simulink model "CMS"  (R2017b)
settings: Solver=FixedStepDiscrete  StartTime=0.0  StopTime=10.0  FixedStep=0.01  RelTol=1e-3  EnableMultiTasking=on
undefined symbols (not defined in the file): ASWTYPE_FALSE, ASWTYPE_TRUE, CcCMS_CANSendDelay_ms, CcCMS_ChrgMaxPackVoltLimt_V, CcCMS_PeakVoltCh_V, CcCMS_PeakVoltDisCh_V, CcSOC_DispSOCHighThrhd_pct, CMS09D_RUNTIME_MS, CMS_CONST0_NUMB, CMS_CONST1000_NUMB, CMS_CONST100_NUMB, CMS_CONST1_NUMB, CMS_CONST2047_NUMB, CMS_CONST2_NUMB, CMS_CONST3_NUMB, CMS_CONST4_NUMB, CMS_CONST5_NUMB, CMS_CONST6_NUMB, CMS_CONST7_NUMB, CMS_CONSTF1_NUMB, Enum_ACCACChrgState, Enum_CMSACChgMode, Enum_CMSBmsSelfChk, Enum_CMSBmsSt, Enum_CMSChgMode, Enum_CMSDCChgMode, Enum_CMSHVBatFltSevrtyStat, Enum_CMSHVConnSt, Enum_CMSPreThmMode, Enum_CMSPreThmReq, Enum_CMSThmPropagation, Enum_CTCCtrCtlConnMode, Enum_CTCCtrCtlState, Enum_DCCDCChrgState, Enum_DCCDCConnSt, Enum_ISOHVIsoFltLevel, Enum_MSMBMUState, Enum_ODPCCState, Enum_VDPPreThmEna
libraries: AIWAYS_Powertrain_BMS_lib x148
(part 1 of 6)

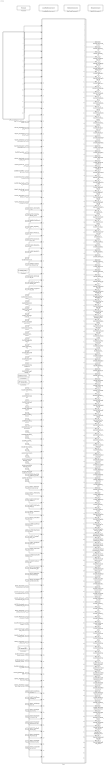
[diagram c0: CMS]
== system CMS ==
  GeCTC_CtrCtlState_enum : Inport
  GbCTC_NegCtlState_flg : Inport  Port=2
  GbCTC_PosCtlState_flg : Inport  Port=3
  GbCTC_DCPosChrgCtlState_flg : Inport  Port=4
  GbCTC_DCNegChrgCtlState_flg : Inport  Port=5
  GcHDP_PackVolt_V : Inport  Port=6
  GbCTC_PreChrgCtlState_flg : Inport  Port=7
  GcHDP_PackCrnt_A : Inport  Port=8
  GbWSM_Kl15WkUpPrs_flg : Inport  Port=9
  GcCDP_MinCellVolt_mV : Inport  Port=10
  GcCDP_MaxCellVolt_mV : Inport  Port=11
  GbACC_ObcChrgCmd_flg : Inport  Port=12
  GcACC_ACChrgVoltRqst_V : Inport  Port=13
  GcACC_ACChrgCrntRqst_A : Inport  Port=14
  GbACC_ACChrgRqst_flg : Inport  Port=15
  GeCTC_CtrCtlConnMode_enum : Inport  Port=16
  GbMSM_SelfCheck_flg : Inport  Port=17
  GcSOC_DispSOC_pct : Inport  Port=18
  GbISP_TFHvilLFlt_flg : Inport  Port=19
  GbFTC_OpenContactor_flg : Inport  Port=20
  GcSOH_PackSOH_pct : Inport  Port=21
  GcSOC_PackSOC_pct : Inport  Port=22
  GcHDP_HallCrnt_A : Inport  Port=23
  GbMSM_SelfChckMaxTiReach_flg : Inport  Port=24
  GbDCC_DCChrgRqst_flg : Inport  Port=25
  GcSOP_DischrgConstPwr_kW : Inport  Port=26
  GcSOP_ChrgConstPwr_kW : Inport  Port=27
  GcISO_HVIsoValue_kohm : Inport  Port=28
  GeODP_ObcCcSt_enum : Inport  Port=29
  GbDCC_DCChrgFinish_flg : Inport  Port=30
  GbACC_ACChrgFinish_flg : Inport  Port=31
  GeACC_ACChrgState_enum : Inport  Port=32
  GeDCC_DCConnSt_enum : Inport  Port=33
  GeLDP_CC2St_enum : Inport  Port=34
  GcCDP_AvgCellTemp_C : Inport  Port=35
  GbISO_IsoForbid_flg : Inport  Port=36
  GcCDP_MaxCellTemp_C : Inport  Port=37
  GcCDP_MinCellTemp_C : Inport  Port=38
  GcDCS_3072ChrgVoltReq_V : Inport  Port=39
  GcDCC_DCChrgCrntRqst_A : Inport  Port=40
  GcLDP_lntWtTemp_C : Inport  Port=41
  GcLDP_OutWtTemp_C : Inport  Port=42
  GcBTM_CoolPwrReq_W : Inport  Port=43
  GcBTM_HeatPwrReq_W : Inport  Port=44
  GeBTM_CoolReq_enum : Inport  Port=45
  GeBTM_HeatReq_enum : Inport  Port=46
  GbODP_V2XDischrgCmd_flg : Inport  Port=47
  GeMSM_BMUState_enum : Inport  Port=48
  GcHDP_FuseVolt_V : Inport  Port=49
  GbADP_DischgReq_flg : Inport  Port=50
  GcHDP_PosCtlVolt_V : Inport  Port=51
  GcCDP_MaxCellVoltNumb_numb : Inport  Port=52
  GcCDP_MinCellVoltNumb_numb : Inport  Port=53
  GcCDP_MaxCellTempNumb_numb : Inport  Port=54
  GcCDP_MinCellTempNumb_numb : Inport  Port=55
  GbWSM_DCWkUpPrs_flg : Inport  Port=56
  GbACC_PreThmObcChrgCmd_flg : Inport  Port=57
  GbACC_PreThmRqst_flg : Inport  Port=58
  GcACC_PreThmCrntRqst_A : Inport  Port=59
  GcACC_PreThmVoltRqst_V : Inport  Port=60
  GbACC_PreHeatPrmt_flg : Inport  Port=61
  GbFTC_PowerDown_flg : Inport  Port=62
  GcBTM_CoolTempReq_C : Inport  Port=63
  GcBTM_HeatTempReq_C : Inport  Port=64
  GcACC_ChrgingTiRem_min : Inport  Port=65
  GcDCC_ChrgingTiRem_min : Inport  Port=66
  GeVDP_PreThmEna_enum : Inport  Port=67
  GcSOP_DischrgPwr_kW : Inport  Port=68
  GcSOP_ChrgPwr_kW : Inport  Port=69
  GbFTC_DischrgPwrLimitLevel3_flg : Inport  Port=70
  GbFTC_RegenPwrLimitLevel3_flg : Inport  Port=71
  GbFTC_DischrgPwrLimitLevel2_flg : Inport  Port=72
  GbFTC_RegenPwrLimitLevel2_flg : Inport  Port=73
  GbFTC_DCChrgCurrLimitLevel2_flg : Inport  Port=74
  GbFTC_ACChrgCurrLimitLevel2_flg : Inport  Port=75
  GbFTC_DischrgPwrLimitLevel1_flg : Inport  Port=76
  GbFTC_RegenPwrLimitLevel1_flg : Inport  Port=77
  GcCDP_MaxBusbarTemp_C : Inport  Port=78
  GcCDP_MinBusbarTemp_C : Inport  Port=79
  GeDCC_DCChrgState_enum : Inport  Port=80
  GeLDP_ChrgGunConnSt_enum : Inport  Port=81
  GbISP_TFThmRnwyfDet_flg : Inport  Port=82
  GcUDS_CellTempNumb_numb : Inport  Port=83
  GcUDS_BusbarTempNumb_numb : Inport  Port=84
  GcUDS_CellVoltNum_numb : Inport  Port=85
  GcUDS_BatEnergy_kWh : Inport  Port=86
  GbACC_HoldTempPrmt_flg : Inport  Port=87
  GbACC_HoldTempObcChrgCmd_flg : Inport  Port=88
  GcACC_HoldTempVoltRqst_V : Inport  Port=89
  GcACC_HoldTempCrntRqst_A : Inport  Port=90
  GbACC_HoldTempRqst_flg : Inport  Port=91
  GbISP_TFIsoResFltLevel2_flg : Inport  Port=92
  GbISP_TFIsoDCResFltLevel2_flg : Inport  Port=93
  GbISP_TFIsoHVoffResFltLevel2_flg : Inport  Port=94
  GbISP_TFIsoResFltLevel1_flg : Inport  Port=95
  GbISP_TFIsoDCResFltLevel1_flg : Inport  Port=96
  GbISP_TFIsoHVoffResFltLevel1_flg : Inport  Port=97
  GbFTC_Level1FltReaction_flg : Inport  Port=98
  CMS : Subsystem
  CMS_Schedule : Stateflow chart  TreatAsAtomicUnit=on
  Constant : Constant  Value=1*ones(112,1)  OutDataTypeStr=boolean
  Constant1 : Constant  Value=25*ones(48,1)  OutDataTypeStr=single
  Constant2 : Constant  Value=25*ones(48,1)  OutDataTypeStr=single
  Constant3 : Constant  Value=4000*ones(112,1)  OutDataTypeStr=uint16
  LoadMptEnvironment : AIWAYS_Powertrain_BMS_lib/Config/LoadMptEnvironment  ProjectName=Comm  SuppierID=NewPlatformUAES
  MptA2LGenerate1 : AIWAYS_Powertrain_BMS_lib/Config/MptA2LGenerate  SystemSampleTime=-1
  MptCodeGenerate1 : AIWAYS_Powertrain_BMS_lib/Config/MptCodeGenerate  SystemSampleTime=-1
  Revision : AIWAYS_Powertrain_BMS_lib/Config/Revision  curVersion='M100C100'  newVersion='M100C100'
  GeCMS_HVConnSt_enum : Outport
  GbCMS_NegCtlSt_flg : Outport  Port=2
  GbCMS_PosCtlSt_flg : Outport  Port=3
  GbCMS_ChrgPosCtlSt_flg : Outport  Port=4
  GbCMS_ChrgNegCtlSt_flg : Outport  Port=5
  GeCMS_RelStuckClosed_enum : Outport  Port=6
  GcCMS_PackVolt_V : Outport  Port=7
  GbCMS_PreChrgCtlSt_flg : Outport  Port=8
  GcCMS_BattCurr_A : Outport  Port=9
  GbCMS_Kl15WkUp_flg : Outport  Port=10
  GbCMS_ThmRunAway_flg : Outport  Port=11
  GcCMS_CoolTempIn_C : Outport  Port=12
  GcCMS_CoolTempOut_C : Outport  Port=13
  GcCMS_CoolPwrReq_W : Outport  Port=14
  GcCMS_HeatPwrReq_W : Outport  Port=15
  GeCMS_CoolReq_enum : Outport  Port=16
  GeCMS_HeatReq_enum : Outport  Port=17
  GcCMS_PeakCurrDisCh_A : Outport  Port=18
  GcCMS_PeakCurrCh_A : Outport  Port=19
  GcCMS_PeakVoltDisCh_V : Outport  Port=20
  GcCMS_PeakVoltCh_V : Outport  Port=21
  GeCMS_Thm_propagat_enum : Outport  Port=22
  GcCMS_ClntTgtTemp_C : Outport  Port=23
  GcCMS_HtTgtTemp_C : Outport  Port=24
  GcCMS_MaxCellVolt_V : Outport  Port=25
  GcCMS_BusbarTempMax_C : Outport  Port=26
  GcCMS_BusbarTempMin_C : Outport  Port=27
  GcCMS_MinCellVolt_V : Outport  Port=28
  GbCMS_ChrgCmd_flg : Outport  Port=29
  GcCMS_ActPwrChrg_Kw : Outport  Port=30
  GcCMS_MaxVoltChrg_V : Outport  Port=31
  GcCMS_ReqVoltChrg_V : Outport  Port=32
  GcCMS_ReqCurrChrg_A : Outport  Port=33
  GbCMS_ObcRdyReq_flg : Outport  Port=34
  GbCMS_DischgCmd_flg : Outport  Port=35
  GeCMS_BmsSt_enum : Outport  Port=36
  GeCMS_BmsSelfChk_enum : Outport  Port=37
  GeCMS_IsoFault_enum : Outport  Port=38
  GcCMS_SocDspl_pct : Outport  Port=39
  GbCMS_HvilOpenFault_flg : Outport  Port=40
  GeCMS_FltLvl_enum : Outport  Port=41
  GeCMS_V2xMod_enum : Outport  Port=42
  GcCMS_ChgSOCset_pct : Outport  Port=43
  GcCMS_BattSoh_pct : Outport  Port=44
  GcCMS_SOCA_pct : Outport  Port=45
  GeCMS_IviDischg_enum : Outport  Port=46
  GcCMS_PackCurLem_A : Outport  Port=47
  GcCMS_BattInVolt_V : Outport  Port=48
  GbCMS_BalSt_flg : Outport  Port=49
  GbCMS_BalVlg_flg : Outport  Port=50
  GbCMS_VcuPwrUpReq_flg : Outport  Port=51
  GbCMS_VcuPwrUpReqVld_flg : Outport  Port=52
  GcCMS_ConstCurrDisChMax_A : Outport  Port=53
  GcCMS_ConstCurrChMax_A : Outport  Port=54
  GbCMS_PwrDownReq_flg : Outport  Port=55
  GbCMS_PwrDownReqVld_flg : Outport  Port=56
  GeCMS_ChrgPreThmMode_enum : Outport  Port=57
  GeCMS_ElockReq_enum : Outport  Port=58
  GeCMS_PreThmReq_enum : Outport  Port=59
  GcCMS_PeakPwrDisCh_Kw : Outport  Port=60
  GcCMS_PeakPwrCh_Kw : Outport  Port=61
  GcCMS_ConstPwrDisCh_Kw : Outport  Port=62
  GcCMS_ConstPwrCh_Kw : Outport  Port=63
  GcCMS_ResIso_Kohm : Outport  Port=64
  GcCMS_ChrgRemTime_Min : Outport  Port=65
  GeCMS_ACPlugCnnt_enum : Outport  Port=66
  GbCMS_BattFull_flg : Outport  Port=67
  GbCMS_WarnLamp_flg : Outport  Port=68
  GbCMS_SerLamp_flg : Outport  Port=69
  GbCMS_TempDiffWarn_flg : Outport  Port=70
  GbCMS_OverChrgWarn_flg : Outport  Port=71
  GbCMS_ConsisWarn_flg : Outport  Port=72
  GbCMS_MishWarn_flg : Outport  Port=73
  GbCMS_SocHopWarn_flg : Outport  Port=74
  GbCMS_SocHighWarn_flg : Outport  Port=75
  GbCMS_SocLowWarn_flg : Outport  Port=76
  GbCMS_OTAModeSt_flg : Outport  Port=77
  GeCMS_AcDcConnBoth_enum : Outport  Port=78
  GbCMS_CellUvFlt_flg : Outport  Port=79
  GbCMS_CellOvFlt_flg : Outport  Port=80
  GbCMS_PackUvFlt_flg : Outport  Port=81
  GbCMS_PackOvFlt_flg : Outport  Port=82
  GbCMS_TempHighWarn_flg : Outport  Port=83
  GcCMS_RealSoc_pct : Outport  Port=84
  GeCMS_DCPlugConn_enum : Outport  Port=85
  GeCMS_ACChgMode_enum : Outport  Port=86
  GeCMS_DCChgMode_enum : Outport  Port=87
  GcCMS_BattTempAvrg_C : Outport  Port=88
  GcCMS_BattNrmEnrg_kwh : Outport  Port=89
  GbCMS_BattTempFault_flg : Outport  Port=90
  GcCMS_BattSoe_kwh : Outport  Port=91
  GbCMS_IsoChkSt_flg : Outport  Port=92
  GcCMS_BattTempMax_C : Outport  Port=93
  GcCMS_BattTempMin_C : Outport  Port=94
  GcCMS_FuseVolt_V : Outport  Port=95
  GcCMS_ChrgAccum_Ah : Outport  Port=96
  GbCMS_DChgStVoltOut_flg : Outport  Port=97
  GcCMS_DChrgVoltReq_V : Outport  Port=98
  GcCMS_DChrgCurrReq_A : Outport  Port=99
  GcCMS_DChrgRchSocLmt_numb : Outport  Port=100
  GcCMS_DChrgRchPackVoltLmt_numb : Outport  Port=101
  GcCMS_DChrgRchCellVoltLmt_numb : Outport  Port=102
  GcCMS_DChrgChrgerActStop_numb : Outport  Port=103
  GcCMS_DChrgBattInsulationErr_numb : Outport  Port=104
  GcCMS_DChrgOutpCnntOvrTempErr_numb : Outport  Port=105
  GcCMS_PcbOvrTempErr_numb : Outport  Port=106
  GcCMS_ChrgCnntErr_numb : Outport  Port=107
  GcCMS_BattOvrTempErr_numb : Outport  Port=108
  GcCMS_MainRelayErr_numb : Outport  Port=109
  GcCMS_CC2ChkVoltErr_numb : Outport  Port=110
  GcCMS_OtherErr_numb : Outport  Port=111
  GcCMS_ChrgCurrAbnrm_numb : Outport  Port=112
  GcCMS_ChrgVoltAbnrm_numb : Outport  Port=113
  GcCMS_CellVoltCnt_numb : Outport  Port=114
  GcCMS_CellVolt1_V : Outport  Port=115
  GcCMS_CellVolt2_V : Outport  Port=116
  GcCMS_CellVolt3_V : Outport  Port=117
  GcCMS_CellVolt4_V : Outport  Port=118
  GcCMS_CellTempCnt_numb : Outport  Port=119
  GcCMS_CellTemp1_C : Outport  Port=120
  GcCMS_CellTemp2_C : Outport  Port=121
  GcCMS_CellTemp3_C : Outport  Port=122
  GcCMS_CellTemp4_C : Outport  Port=123
  GcCMS_CellTemp5_C : Outport  Port=124
  GcCMS_CellTemp6_C : Outport  Port=125
  GcCMS_CellTemp7_C : Outport  Port=126
  GcCMS_MaxCellVoltNumb_numb : Outport  Port=127
  GcCMS_MinCellVoltNumb_numb : Outport  Port=128
  GcCMS_MaxCellTempNumb_numb : Outport  Port=129
  GcCMS_MinCellTempNumb_numb : Outport  Port=130
  GcCMS_MaxVoltNumb_numb : Outport  Port=131
  GcCMS_MinVoltNumb_numb : Outport  Port=132
  GcCMS_MaxTempNumb_numb : Outport  Port=133
  GcCMS_MinTempNumb_numb : Outport  Port=134
  GeCMS_ChgMode_enum : Outport  Port=135
  GeCMS_DChrgModeDebug_enum : Outport  Port=136
  GbCMS_DChrgWkUp_flg : Outport  Port=137
  GeCMS_EvccMode_enum : Outport  Port=138
  GeCMS_AChrgObsr_enum : Outport  Port=139
  GeCMS_PreThmObsvr_enum : Outport  Port=140
  GbCMS_StartCanSend_flg : Outport  Port=141
  GeCMS_AppChgMode_enum : Outport  Port=142
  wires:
  CMS/1(GeCMS_HVConnSt_enum) -> GeCMS_HVConnSt_enum/1
  CMS/2(GbCMS_NegCtlSt_flg) -> GbCMS_NegCtlSt_flg/1
  CMS/3(GbCMS_PosCtlSt_flg) -> GbCMS_PosCtlSt_flg/1
  CMS/4(GbCMS_ChrgPosCtlSt_flg) -> GbCMS_ChrgPosCtlSt_flg/1
  CMS/5(GbCMS_ChrgNegCtlSt_flg) -> GbCMS_ChrgNegCtlSt_flg/1
  CMS/6(GeCMS_RelStuckClosed_enum) -> GeCMS_RelStuckClosed_enum/1
  CMS/7(GcCMS_PackVolt_V) -> GcCMS_PackVolt_V/1
  CMS/8(GbCMS_PreChrgCtlSt_flg) -> GbCMS_PreChrgCtlSt_flg/1
  CMS/9(GcCMS_BattCurr_A) -> GcCMS_BattCurr_A/1
  CMS/10(GbCMS_Kl15WkUp_flg) -> GbCMS_Kl15WkUp_flg/1
  CMS/11(GbCMS_ThmRunAway_flg) -> GbCMS_ThmRunAway_flg/1
  CMS/12(GcCMS_CoolTempIn_C) -> GcCMS_CoolTempIn_C/1
  CMS/13(GcCMS_CoolTempOut_C) -> GcCMS_CoolTempOut_C/1
  CMS/14(GcCMS_CoolPwrReq_W) -> GcCMS_CoolPwrReq_W/1
  CMS/15(GcCMS_HeatPwrReq_W) -> GcCMS_HeatPwrReq_W/1
  CMS/16(GeCMS_CoolReq_enum) -> GeCMS_CoolReq_enum/1
  CMS/17(GeCMS_HeatReq_enum) -> GeCMS_HeatReq_enum/1
  CMS/18(GcCMS_PeakCurrDisCh_A) -> GcCMS_PeakCurrDisCh_A/1
  CMS/19(GcCMS_PeakCurrCh_A) -> GcCMS_PeakCurrCh_A/1
  CMS/20(GcCMS_PeakVoltDisCh_V) -> GcCMS_PeakVoltDisCh_V/1
  CMS/21(GcCMS_PeakVoltCh_V) -> GcCMS_PeakVoltCh_V/1
  CMS/140(GeCMS_Thm_propagat_enum) -> GeCMS_Thm_propagat_enum/1
  CMS/22(GcCMS_ClntTgtTemp_C) -> GcCMS_ClntTgtTemp_C/1
  CMS/23(GcCMS_HtTgtTemp_C) -> GcCMS_HtTgtTemp_C/1
  CMS/24(GcCMS_MaxCellVolt_V) -> GcCMS_MaxCellVolt_V/1
  CMS/25(GcCMS_BusbarTempMax_C) -> GcCMS_BusbarTempMax_C/1
  CMS/26(GcCMS_BusbarTempMin_C) -> GcCMS_BusbarTempMin_C/1
  CMS/27(GcCMS_MinCellVolt_V) -> GcCMS_MinCellVolt_V/1
  CMS/28(GbCMS_ChrgCmd_flg) -> GbCMS_ChrgCmd_flg/1
  CMS/29(GcCMS_ActPwrChrg_Kw) -> GcCMS_ActPwrChrg_Kw/1
  CMS/30(GcCMS_MaxVoltChrg_V) -> GcCMS_MaxVoltChrg_V/1
  CMS/31(GcCMS_ReqVoltChrg_V) -> GcCMS_ReqVoltChrg_V/1
  CMS/32(GcCMS_ReqCurrChrg_A) -> GcCMS_ReqCurrChrg_A/1
  CMS/33(GbCMS_ObcRdyReq_flg) -> GbCMS_ObcRdyReq_flg/1
  CMS/34(GbCMS_DischgCmd_flg) -> GbCMS_DischgCmd_flg/1
  CMS/35(GeCMS_BmsSt_enum) -> GeCMS_BmsSt_enum/1
  CMS/36(GeCMS_BmsSelfChk_enum) -> GeCMS_BmsSelfChk_enum/1
  CMS/37(GeCMS_IsoFault_enum) -> GeCMS_IsoFault_enum/1
  CMS/38(GcCMS_SocDspl_pct) -> GcCMS_SocDspl_pct/1
  CMS/39(GbCMS_HvilOpenFault_flg) -> GbCMS_HvilOpenFault_flg/1
  CMS/40(GeCMS_FltLvl_enum) -> GeCMS_FltLvl_enum/1
  CMS/41(GeCMS_V2xMod_enum) -> GeCMS_V2xMod_enum/1
  CMS/42(GcCMS_ChgSOCset_pct) -> GcCMS_ChgSOCset_pct/1
  CMS/43(GcCMS_BattSoh_pct) -> GcCMS_BattSoh_pct/1
  CMS/44(GcCMS_SOCA_pct) -> GcCMS_SOCA_pct/1
  CMS/45(GeCMS_IviDischg_enum) -> GeCMS_IviDischg_enum/1
  CMS/46(GcCMS_PackCurLem_A) -> GcCMS_PackCurLem_A/1
  CMS/47(GcCMS_BattInVolt_V) -> GcCMS_BattInVolt_V/1
  CMS/48(GbCMS_BalSt_flg) -> GbCMS_BalSt_flg/1
  CMS/49(GbCMS_BalVlg_flg) -> GbCMS_BalVlg_flg/1
  CMS/50(GbCMS_VcuPwrUpReq_flg) -> GbCMS_VcuPwrUpReq_flg/1
  CMS/51(GbCMS_VcuPwrUpReqVld_flg) -> GbCMS_VcuPwrUpReqVld_flg/1
  CMS/52(GcCMS_ConstCurrDisChMax_A) -> GcCMS_ConstCurrDisChMax_A/1
  CMS/53(GcCMS_ConstCurrChMax_A) -> GcCMS_ConstCurrChMax_A/1
  CMS/54(GbCMS_PwrDownReq_flg) -> GbCMS_PwrDownReq_flg/1
  CMS/55(GbCMS_PwrDownReqVld_flg) -> GbCMS_PwrDownReqVld_flg/1
  CMS/56(GeCMS_ChrgPreThmMode_enum) -> GeCMS_ChrgPreThmMode_enum/1
  CMS/57(GeCMS_ElockReq_enum) -> GeCMS_ElockReq_enum/1
  CMS/58(GeCMS_PreThmReq_enum) -> GeCMS_PreThmReq_enum/1
  CMS/59(GcCMS_PeakPwrDisCh_Kw) -> GcCMS_PeakPwrDisCh_Kw/1
  CMS/60(GcCMS_PeakPwrCh_Kw) -> GcCMS_PeakPwrCh_Kw/1
  CMS/61(GcCMS_ConstPwrDisCh_Kw) -> GcCMS_ConstPwrDisCh_Kw/1
  CMS/62(GcCMS_ConstPwrCh_Kw) -> GcCMS_ConstPwrCh_Kw/1
  CMS/63(GcCMS_ResIso_Kohm) -> GcCMS_ResIso_Kohm/1
  CMS/64(GcCMS_ChrgRemTime_Min) -> GcCMS_ChrgRemTime_Min/1
  CMS/65(GeCMS_ACPlugCnnt_enum) -> GeCMS_ACPlugCnnt_enum/1
  CMS/66(GbCMS_BattFull_flg) -> GbCMS_BattFull_flg/1
  CMS/67(GbCMS_WarnLamp_flg) -> GbCMS_WarnLamp_flg/1
  CMS/68(GbCMS_SerLamp_flg) -> GbCMS_SerLamp_flg/1
  CMS/69(GbCMS_TempDiffWarn_flg) -> GbCMS_TempDiffWarn_flg/1
  CMS/70(GbCMS_OverChrgWarn_flg) -> GbCMS_OverChrgWarn_flg/1
  CMS/71(GbCMS_ConsisWarn_flg) -> GbCMS_ConsisWarn_flg/1
  CMS/72(GbCMS_MishWarn_flg) -> GbCMS_MishWarn_flg/1
  CMS/73(GbCMS_SocHopWarn_flg) -> GbCMS_SocHopWarn_flg/1
  CMS/74(GbCMS_SocHighWarn_flg) -> GbCMS_SocHighWarn_flg/1
  CMS/75(GbCMS_SocLowWarn_flg) -> GbCMS_SocLowWarn_flg/1
  CMS/76(GbCMS_OTAModeSt_flg) -> GbCMS_OTAModeSt_flg/1
  CMS/77(GeCMS_AcDcConnBoth_enum) -> GeCMS_AcDcConnBoth_enum/1
  CMS/78(GbCMS_CellUvFlt_flg) -> GbCMS_CellUvFlt_flg/1
  CMS/79(GbCMS_CellOvFlt_flg) -> GbCMS_CellOvFlt_flg/1
  CMS/80(GbCMS_PackUvFlt_flg) -> GbCMS_PackUvFlt_flg/1
  CMS/81(GbCMS_PackOvFlt_flg) -> GbCMS_PackOvFlt_flg/1
  CMS/82(GbCMS_TempHighWarn_flg) -> GbCMS_TempHighWarn_flg/1
  CMS/83(GcCMS_RealSoc_pct) -> GcCMS_RealSoc_pct/1
  CMS/84(GeCMS_DCPlugConn_enum) -> GeCMS_DCPlugConn_enum/1
  CMS/85(GeCMS_ACChgMode_enum) -> GeCMS_ACChgMode_enum/1
  CMS/86(GeCMS_DCChgMode_enum) -> GeCMS_DCChgMode_enum/1
  CMS/87(GcCMS_BattTempAvrg_C) -> GcCMS_BattTempAvrg_C/1
  CMS/88(GcCMS_BattNrmEnrg_kwh) -> GcCMS_BattNrmEnrg_kwh/1
  CMS/89(GbCMS_BattTempFault_flg) -> GbCMS_BattTempFault_flg/1
  CMS/90(GcCMS_BattSoe_kwh) -> GcCMS_BattSoe_kwh/1
  CMS/91(GbCMS_IsoChkSt_flg) -> GbCMS_IsoChkSt_flg/1
  CMS/92(GcCMS_BattTempMax_C) -> GcCMS_BattTempMax_C/1
  CMS/93(GcCMS_BattTempMin_C) -> GcCMS_BattTempMin_C/1
  CMS/94(GcCMS_FuseVolt_V) -> GcCMS_FuseVolt_V/1
  CMS/95(GcCMS_ChrgAccum_Ah) -> GcCMS_ChrgAccum_Ah/1
  CMS/96(GbCMS_DChgStVoltOut_flg) -> GbCMS_DChgStVoltOut_flg/1
  CMS/97(GcCMS_DChrgVoltReq_V) -> GcCMS_DChrgVoltReq_V/1
  CMS/98(GcCMS_DChrgCurrReq_A) -> GcCMS_DChrgCurrReq_A/1
  CMS/99(GcCMS_DChrgRchSocLmt_numb) -> GcCMS_DChrgRchSocLmt_numb/1
  CMS/100(GcCMS_DChrgRchPackVoltLmt_numb) -> GcCMS_DChrgRchPackVoltLmt_numb/1
  CMS/101(GcCMS_DChrgRchCellVoltLmt_numb) -> GcCMS_DChrgRchCellVoltLmt_numb/1
  CMS/102(GcCMS_DChrgChrgerActStop_numb) -> GcCMS_DChrgChrgerActStop_numb/1
  CMS/103(GcCMS_DChrgBattInsulationErr_numb) -> GcCMS_DChrgBattInsulationErr_numb/1
  CMS/104(GcCMS_DChrgOutpCnntOvrTempErr_numb) -> GcCMS_DChrgOutpCnntOvrTempErr_numb/1
  CMS/105(GcCMS_PcbOvrTempErr_numb) -> GcCMS_PcbOvrTempErr_numb/1
  CMS/106(GcCMS_ChrgCnntErr_numb) -> GcCMS_ChrgCnntErr_numb/1
  CMS/107(GcCMS_BattOvrTempErr_numb) -> GcCMS_BattOvrTempErr_numb/1
  CMS/108(GcCMS_MainRelayErr_numb) -> GcCMS_MainRelayErr_numb/1
  CMS/109(GcCMS_CC2ChkVoltErr_numb) -> GcCMS_CC2ChkVoltErr_numb/1
  CMS/110(GcCMS_OtherErr_numb) -> GcCMS_OtherErr_numb/1
  CMS/111(GcCMS_ChrgCurrAbnrm_numb) -> GcCMS_ChrgCurrAbnrm_numb/1
  CMS/112(GcCMS_ChrgVoltAbnrm_numb) -> GcCMS_ChrgVoltAbnrm_numb/1
  CMS/113(GcCMS_CellVoltCnt_numb) -> GcCMS_CellVoltCnt_numb/1
  CMS/114(GcCMS_CellVolt1_V) -> GcCMS_CellVolt1_V/1
  CMS/115(GcCMS_CellVolt2_V) -> GcCMS_CellVolt2_V/1
  CMS/116(GcCMS_CellVolt3_V) -> GcCMS_CellVolt3_V/1
  CMS/117(GcCMS_CellVolt4_V) -> GcCMS_CellVolt4_V/1
  CMS/118(GcCMS_CellTempCnt_numb) -> GcCMS_CellTempCnt_numb/1
  CMS/119(GcCMS_CellTemp1_C) -> GcCMS_CellTemp1_C/1
  CMS/120(GcCMS_CellTemp2_C) -> GcCMS_CellTemp2_C/1
  CMS/121(GcCMS_CellTemp3_C) -> GcCMS_CellTemp3_C/1
  CMS/122(GcCMS_CellTemp4_C) -> GcCMS_CellTemp4_C/1
  CMS/123(GcCMS_CellTemp5_C) -> GcCMS_CellTemp5_C/1
  CMS/124(GcCMS_CellTemp6_C) -> GcCMS_CellTemp6_C/1
  CMS/125(GcCMS_CellTemp7_C) -> GcCMS_CellTemp7_C/1
  GeCTC_CtrCtlState_enum/1 -> CMS/15(GeCTC_CtrCtlState_enum)
  GbCTC_NegCtlState_flg/1 -> CMS/16(GbCTC_NegCtlState_flg)
  GbCTC_PosCtlState_flg/1 -> CMS/17(GbCTC_PosCtlState_flg)
  GbCTC_DCPosChrgCtlState_flg/1 -> CMS/18(GbCTC_DCPosChrgCtlState_flg)
  GbCTC_DCNegChrgCtlState_flg/1 -> CMS/19(GbCTC_DCNegChrgCtlState_flg)
  GcHDP_PackVolt_V/1 -> CMS/20(GcHDP_PackVolt_V)
  GbCTC_PreChrgCtlState_flg/1 -> CMS/21(GbCTC_PreChrgCtlState_flg)
  GcHDP_PackCrnt_A/1 -> CMS/22(GcHDP_PackCrnt_A)
  GbWSM_Kl15WkUpPrs_flg/1 -> CMS/23(GbWSM_Kl15WkUpPrs_flg)
  GcCDP_MinCellVolt_mV/1 -> CMS/24(GcCDP_MinCellVolt_mV)
  GcCDP_MaxCellVolt_mV/1 -> CMS/25(GcCDP_MaxCellVolt_mV)
  GbACC_ObcChrgCmd_flg/1 -> CMS/26(GbACC_ObcChrgCmd_flg)
  GcACC_ACChrgVoltRqst_V/1 -> CMS/27(GcACC_ACChrgVoltRqst_V)
  GcACC_ACChrgCrntRqst_A/1 -> CMS/28(GcACC_ACChrgCrntRqst_A)
  GbACC_ACChrgRqst_flg/1 -> CMS/29(GbACC_ACChrgRqst_flg)
  GeCTC_CtrCtlConnMode_enum/1 -> CMS/30(GeCTC_CtrCtlConnMode_enum)
  GbMSM_SelfCheck_flg/1 -> CMS/31(GbMSM_SelfCheck_flg)
  GcSOC_DispSOC_pct/1 -> CMS/32(GcSOC_DispSOC_pct)
  GbISP_TFHvilLFlt_flg/1 -> CMS/33(GbISP_TFHvilLFlt_flg)
  GbFTC_OpenContactor_flg/1 -> CMS/34(GbFTC_OpenContactor_flg)
  GcSOH_PackSOH_pct/1 -> CMS/35(GcSOH_PackSOH_pct)
  GcSOC_PackSOC_pct/1 -> CMS/36(GcSOC_PackSOC_pct)
  GcHDP_HallCrnt_A/1 -> CMS/37(GcHDP_HallCrnt_A)
  GbMSM_SelfChckMaxTiReach_flg/1 -> CMS/38(GbMSM_SelfChckMaxTiReach_flg)
  Constant/1 -> CMS/39(GaCDP_CellBalc_flg)
  GbDCC_DCChrgRqst_flg/1 -> CMS/40(GbDCC_DCChrgRqst_flg)
  GcSOP_DischrgConstPwr_kW/1 -> CMS/41(GcSOP_DischrgConstPwr_kW)
  GcSOP_ChrgConstPwr_kW/1 -> CMS/42(GcSOP_ChrgConstPwr_kW)
  GcISO_HVIsoValue_kohm/1 -> CMS/43(GcISO_HVIsoValue_kohm)
  GeODP_ObcCcSt_enum/1 -> CMS/44(GeODP_ObcCcSt_enum)
  GbDCC_DCChrgFinish_flg/1 -> CMS/45(GbDCC_DCChrgFinish_flg)
  GbACC_ACChrgFinish_flg/1 -> CMS/46(GbACC_ACChrgFinish_flg)
  GeACC_ACChrgState_enum/1 -> CMS/47(GeACC_ACChrgState_enum)
  GeDCC_DCConnSt_enum/1 -> CMS/48(GeDCC_DCConnSt_enum)
  GeLDP_CC2St_enum/1 -> CMS/49(GeLDP_CC2St_enum)
  GcCDP_AvgCellTemp_C/1 -> CMS/50(GcCDP_AvgCellTemp_C)
  GbISO_IsoForbid_flg/1 -> CMS/51(GbISO_IsoForbid_flg)
  GcCDP_MaxCellTemp_C/1 -> CMS/52(GcCDP_MaxCellTemp_C)
  GcCDP_MinCellTemp_C/1 -> CMS/53(GcCDP_MinCellTemp_C)
  GcDCS_3072ChrgVoltReq_V/1 -> CMS/54(GcDCS_3072ChrgVoltReq_V)
  GcDCC_DCChrgCrntRqst_A/1 -> CMS/55(GcDCC_DCChrgCrntRqst_A)
  Constant3/1 -> CMS/56(GaCDP_CellVolt_mV)
  Constant1/1 -> CMS/57(GaCDP_CellTemp_C)
  GcLDP_lntWtTemp_C/1 -> CMS/58(GcLDP_lntWtTemp_C)
  GcLDP_OutWtTemp_C/1 -> CMS/59(GcLDP_OutWtTemp_C)
  GcBTM_CoolPwrReq_W/1 -> CMS/60(GcBTM_CoolPwrReq_W)
  GcBTM_HeatPwrReq_W/1 -> CMS/61(GcBTM_HeatPwrReq_W)
  GeBTM_CoolReq_enum/1 -> CMS/62(GeBTM_CoolReq_enum)
  GeBTM_HeatReq_enum/1 -> CMS/63(GeBTM_HeatReq_enum)
  GbODP_V2XDischrgCmd_flg/1 -> CMS/64(GbODP_V2XDischrgCmd_flg)
  GeMSM_BMUState_enum/1 -> CMS/65(GeMSM_BMUState_enum)
  GcHDP_FuseVolt_V/1 -> CMS/66(GcHDP_FuseVolt_V)
  GbADP_DischgReq_flg/1 -> CMS/67(GbADP_DischgReq_flg)
  GcHDP_PosCtlVolt_V/1 -> CMS/68(GcHDP_PosCtlVolt_V)
  GcCDP_MaxCellVoltNumb_numb/1 -> CMS/69(GcCDP_MaxCellVoltNumb_numb)
  GbWSM_DCWkUpPrs_flg/1 -> CMS/73(GbWSM_DCWkUpPrs_flg)
  GcCDP_MinCellTempNumb_numb/1 -> CMS/72(GcCDP_MinCellTempNumb_numb)
  GcCDP_MaxCellTempNumb_numb/1 -> CMS/71(GcCDP_MaxCellTempNumb_numb)
  GcCDP_MinCellVoltNumb_numb/1 -> CMS/70(GcCDP_MinCellVoltNumb_numb)
  CMS/126(GcCMS_MaxCellVoltNumb_numb) -> GcCMS_MaxCellVoltNumb_numb/1
  CMS/127(GcCMS_MinCellVoltNumb_numb) -> GcCMS_MinCellVoltNumb_numb/1
  CMS/128(GcCMS_MaxCellTempNumb_numb) -> GcCMS_MaxCellTempNumb_numb/1
  CMS/130(GcCMS_MaxVoltNumb_numb) -> GcCMS_MaxVoltNumb_numb/1
  CMS/129(GcCMS_MinCellTempNumb_numb) -> GcCMS_MinCellTempNumb_numb/1
  CMS/131(GcCMS_MinVoltNumb_numb) -> GcCMS_MinVoltNumb_numb/1
  CMS/132(GcCMS_MaxTempNumb_numb) -> GcCMS_MaxTempNumb_numb/1
  CMS/133(GcCMS_MinTempNumb_numb) -> GcCMS_MinTempNumb_numb/1
  CMS/134(GeCMS_ChgMode_enum) -> GeCMS_ChgMode_enum/1
  CMS/135(GeCMS_DChrgModeDebug_enum) -> GeCMS_DChrgModeDebug_enum/1
  CMS/136(GbCMS_DChrgWkUp_flg) -> GbCMS_DChrgWkUp_flg/1
  CMS/137(GeCMS_EvccMode_enum) -> GeCMS_EvccMode_enum/1
  CMS/138(GeCMS_AChrgObsr_enum) -> GeCMS_AChrgObsr_enum/1
  CMS/139(GeCMS_PreThmObsvr_enum) -> GeCMS_PreThmObsvr_enum/1
  GbACC_PreThmObcChrgCmd_flg/1 -> CMS/74(GbACC_PreThmObcChrgCmd_flg)
  GcACC_PreThmCrntRqst_A/1 -> CMS/76(GcACC_PreThmCrntRqst_A)
  GcACC_PreThmVoltRqst_V/1 -> CMS/77(GcACC_PreThmVoltRqst_V)
  GbACC_PreHeatPrmt_flg/1 -> CMS/78(GbACC_PreHeatPrmt_flg)
  GbACC_PreThmRqst_flg/1 -> CMS/75(GbACC_PreThmRqst_flg)
  GbFTC_PowerDown_flg/1 -> CMS/79(GbFTC_PowerDown_flg)
  GcBTM_CoolTempReq_C/1 -> CMS/80(GcBTM_CoolTempReq_C)
  GcBTM_HeatTempReq_C/1 -> CMS/81(GcBTM_HeatTempReq_C)
  GcACC_ChrgingTiRem_min/1 -> CMS/82(GcACC_ChrgingTiRem_min)
  GcDCC_ChrgingTiRem_min/1 -> CMS/83(GcDCC_ChrgingTiRem_min)
  GeVDP_PreThmEna_enum/1 -> CMS/84(GeVDP_PreThmEna_enum)
  GcSOP_DischrgPwr_kW/1 -> CMS/85(GcSOP_DischrgPwr_kW)
  GcSOP_ChrgPwr_kW/1 -> CMS/86(GcSOP_ChrgPwr_kW)
  GbFTC_DischrgPwrLimitLevel3_flg/1 -> CMS/87(GbFTC_DischrgPwrLimitLevel3_flg)
  GbFTC_RegenPwrLimitLevel3_flg/1 -> CMS/88(GbFTC_RegenPwrLimitLevel3_flg)
  GbFTC_DischrgPwrLimitLevel2_flg/1 -> CMS/89(GbFTC_DischrgPwrLimitLevel2_flg)
  GbFTC_RegenPwrLimitLevel2_flg/1 -> CMS/90(GbFTC_RegenPwrLimitLevel2_flg)
  GbFTC_DCChrgCurrLimitLevel2_flg/1 -> CMS/91(GbFTC_DCChrgCurrLimitLevel2_flg)
  GbFTC_ACChrgCurrLimitLevel2_flg/1 -> CMS/92(GbFTC_ACChrgCurrLimitLevel2_flg)
  GbFTC_DischrgPwrLimitLevel1_flg/1 -> CMS/93(GbFTC_DischrgPwrLimitLevel1_flg)
  GbFTC_RegenPwrLimitLevel1_flg/1 -> CMS/94(GbFTC_RegenPwrLimitLevel1_flg)
  GcCDP_MaxBusbarTemp_C/1 -> CMS/95(GcCDP_MaxBusbarTemp_C)
  GcCDP_MinBusbarTemp_C/1 -> CMS/96(GcCDP_MinBusbarTemp_C)
  GeDCC_DCChrgState_enum/1 -> CMS/97(GeDCC_DCChrgState_enum)
  GeLDP_ChrgGunConnSt_enum/1 -> CMS/98(GeLDP_ChrgGunConnSt_enum)
  GbISP_TFThmRnwyfDet_flg/1 -> CMS/99(GbISP_TFThmRnwyfDet_flg)
  CMS/141(GbCMS_StartCanSend_flg) -> GbCMS_StartCanSend_flg/1
  Constant2/1 -> CMS/100(GaCDP_BusbarTemp_C)
  GcUDS_BusbarTempNumb_numb/1 -> CMS/102(GcUDS_BusbarTempNumb_numb)
  GcUDS_CellTempNumb_numb/1 -> CMS/101(GcUDS_CellTempNumb_numb)
  GcUDS_CellVoltNum_numb/1 -> CMS/103(GcUDS_CellVoltNum_numb)
  GcUDS_BatEnergy_kWh/1 -> CMS/104(GcUDS_BatEnergy_kWh)
  GbACC_HoldTempPrmt_flg/1 -> CMS/105(GbACC_HoldTempPrmt_flg)
  GbACC_HoldTempObcChrgCmd_flg/1 -> CMS/106(GbACC_HoldTempObcChrgCmd_flg)
  GbACC_HoldTempRqst_flg/1 -> CMS/109(GbACC_HoldTempRqst_flg)
  GcACC_HoldTempCrntRqst_A/1 -> CMS/108(GcACC_HoldTempCrntRqst_A)
  GcACC_HoldTempVoltRqst_V/1 -> CMS/107(GcACC_HoldTempVoltRqst_V)
  CMS/142(GeCMS_AppChgMode_enum) -> GeCMS_AppChgMode_enum/1
  GbISP_TFIsoResFltLevel2_flg/1 -> CMS/110(GbISP_TFIsoResFltLevel2_flg)
  GbISP_TFIsoDCResFltLevel2_flg/1 -> CMS/111(GbISP_TFIsoDCResFltLevel2_flg)
  GbISP_TFIsoHVoffResFltLevel2_flg/1 -> CMS/112(GbISP_TFIsoHVoffResFltLevel2_flg)
  GbISP_TFIsoResFltLevel1_flg/1 -> CMS/113(GbISP_TFIsoResFltLevel1_flg)
  GbISP_TFIsoDCResFltLevel1_flg/1 -> CMS/114(GbISP_TFIsoDCResFltLevel1_flg)
  GbISP_TFIsoHVoffResFltLevel1_flg/1 -> CMS/115(GbISP_TFIsoHVoffResFltLevel1_flg)
  GbFTC_Level1FltReaction_flg/1 -> CMS/116(GbFTC_Level1FltReaction_flg)
  CMS_Schedule/1(CMS_09D_10ms()) -> CMS/1(CMS_09D_10ms)
  CMS_Schedule/2(CMS_2C0_100ms()) -> CMS/2(CMS_2C0_100ms)
  CMS_Schedule/3(CMS_2C2_100ms()) -> CMS/3(CMS_2C2_100ms)
  CMS_Schedule/4(CMS_2C3_100ms()) -> CMS/4(CMS_2C3_100ms)
  CMS_Schedule/6(CMS_2C8_100ms()) -> CMS/6(CMS_2C8_100ms)
  CMS_Schedule/5(CMS_2C7_100ms()) -> CMS/5(CMS_2C7_100ms)
  CMS_Schedule/7(CMS_2CA_100ms()) -> CMS/7(CMS_2CA_100ms)
  CMS_Schedule/8(CMS_2CD_100ms()) -> CMS/8(CMS_2CD_100ms)
  CMS_Schedule/9(CMS_2CE_100ms()) -> CMS/9(CMS_2CE_100ms)
  CMS_Schedule/10(CMS_2CF_100ms()) -> CMS/10(CMS_2CF_100ms)
  CMS_Schedule/11(CMS_3B0_1000ms()) -> CMS/11(CMS_3B0_1000ms)
  CMS_Schedule/12(CMS_3E0_20ms()) -> CMS/12(CMS_3E0_20ms)
  CMS_Schedule/13(CMS_3E1_100ms()) -> CMS/13(CMS_3E1_100ms)
  CMS_Schedule/14(CMS_318_500ms()) -> CMS/14(CMS_318_500ms)
